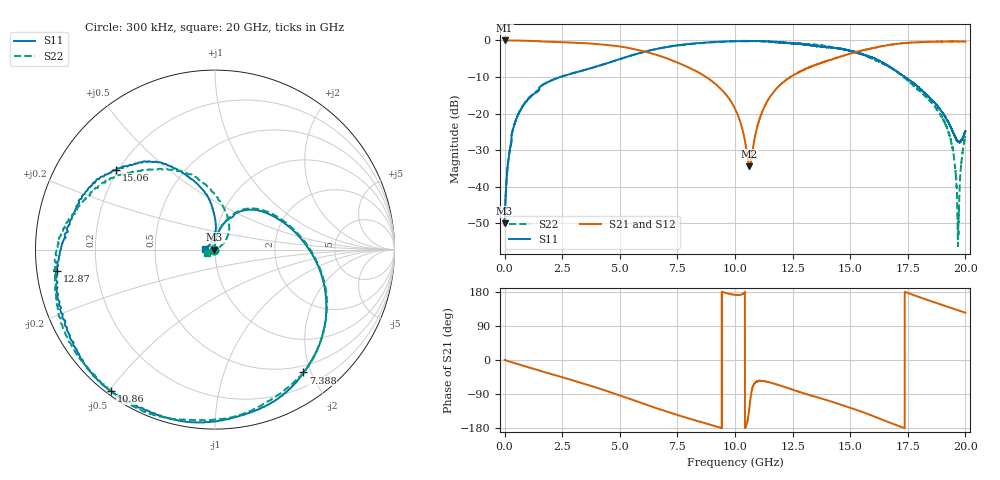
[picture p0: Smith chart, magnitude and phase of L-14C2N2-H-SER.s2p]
!{L-14C2N2}
!Johanson Technology Inc.
!www.johansontechnology.com
!Test Board Conditions:
!Substrate Type  RO4350B
!Substrate Thickness  20 mil
!Substrate Dk  3.66
!TL Type: GCPW
!TL Trace Width  36 mil
!TL Gap  12 mil
!Electrode orientation  Horizontal
!DUT TOPOLOGY	SERIES
!Mounting Pad LxW  26x36 mil
! Created Sun Jun 20 12:54:56 2021
# hz S ma R 50
! 2 Port Network Data from SP1.SP block
! freq  magS11  angS11  magS21  angS21  magS12  angS12  magS22  angS22
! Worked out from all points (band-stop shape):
!   20001 points, 300 kHz to 20 GHz, reference 50 ohm
!   highest |S21| = -0.02 dB at 300 kHz (marker M1); lowest = -34.5 dB at 10.63 GHz (marker M2)
!   |S21| within 3 dB of the highest: start of sweep to 6.056 GHz; 15.36 GHz to end of sweep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
!   lowest |S11| = -50.0 dB at 300 kHz (marker M3), VSWR 1.01, Z = 49.7 + j0.0361 ohm
!   |S11| at or under -10 dB: start of sweep to 2.429 GHz; 17.38 GHz to end of sweep
!   |S22| runs from -56.3 to -0.1 dB; largest |S21 - S12| = 0.017
!   S11 on the Smith chart (normalised r, x): 300 kHz: 0.99, +0.00; 7.388 GHz: 0.40, -1.89; 10.86 GHz: 0.01, -0.51; 12.87 GHz: 0.06, -0.07; 15.06 GHz: 0.19, +0.34; 20 GHz: 0.89, +0.00
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300000  0.003176 173.4  0.9978 -0.0  0.9958 -0.0  0.002909 179.5
1.443e8  0.02036 95.4  0.9968 -2.6  0.9971 -2.7  0.02114 94.9
2.793e8  0.03848 88.9  0.9963 -5.1  0.9965 -5.1  0.03947 89.0
6.973e8  0.1121 77.2  0.992 -13.1  0.992 -13.1  0.1141 77.7
1.6073e9  0.2406 58.9  0.9671 -29.8  0.9671 -29.8  0.2425 59.9
3.3343e9  0.3829 27.7  0.9195 -60.6  0.9199 -60.5  0.3836 30.0
4.9293e9  0.5454 -3.4  0.8311 -92.2  0.8299 -92.0  0.5458 -2.5
6.6673e9  0.7719 -39.7  0.6232 -128.8  0.6202 -128.5  0.7718 -39.7
7.3883e9  0.8433 -54.3  0.5158 -142.8  0.5159 -142.7  0.8448 -54.1
9.0933e9  0.9515 -87.1  0.2628 -173.9  0.2656 -174.0  0.9431 -88.0
1.00003e10  0.975 -106.4  0.1169 172.0  0.1173 172.1  0.9766 -106.7
1.06293e10  0.9755 -121.4  0.01891 -123.1  0.01933 -124.4  0.9851 -119.8
1.08573e10  0.9782 -126.3  0.04647 -60.9  0.04717 -61.1  0.98 -125.1
1.15463e10  0.9587 -141.9  0.1735 -59.7  0.1754 -59.6  0.9653 -142.4
1.28673e10  0.8897 -172.3  0.3827 -85.7  0.3843 -86.1  0.9046 -172.5
1.33343e10  0.8529 177.7  0.4432 -94.2  0.4408 -94.8  0.8787 178.9
1.50613e10  0.7081 141.2  0.6655 -127.5  0.6611 -127.2  0.7195 148.2
1.66673e10  0.4446 111.2  0.8662 -164.1  0.8682 -163.1  0.4424 108.2
1.90233e10  0.1013 88.4  0.9648 144.6  0.9645 144.7  0.08457 42.0
1.94183e10  0.06029 100.6  0.9674 136.7  0.9684 136.5  0.03635 30.9
1.96743e10  0.04188 130.3  0.9681 131.4  0.968 131.4  0.002089 -31.3
2e10  0.05712 179.1  0.9668 124.7  0.9622 124.5  0.0492 -157.4
